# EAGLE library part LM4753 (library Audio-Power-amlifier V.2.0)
The LM4753 is a stereo audio amplifier capable of delivering 10W/channel at 10% distortion into a 8W load. The power amp has an internally set gain of 30 dB. A 0V–5V DC controlled volume block provides 80 dB of attenuation from input to line-out. Line outputs are available after the volume control for signal routing.
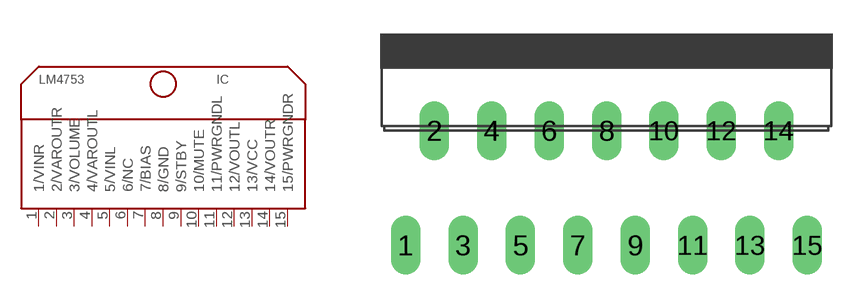
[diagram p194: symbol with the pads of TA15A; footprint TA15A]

Designator prefix IC

## LM4753  [TA15A]
1  1/VINR  in
2  2/VAROUTR  out
3  3/VOLUME  in
4  4/VAROUTL  out
5  5/VINL  in
6  6/NC  nc
7  7/BIAS
8  8/GND  pwr
9  9/STBY  in
10  10/MUTE  in
11  11/PWRGNDL  pwr
12  12/VOUTL  out
13  13/VCC  pwr
14  14/VOUTR  out
15  15/PWRGNDR  pwr

## Footprint TA15A (pad centres in mm)
TA15A www.national.com
drill 0.8 long: 1 -8.89,-5.08; 2 -7.62,0; 3 -6.35,-5.08; 4 -5.08,0; 5 -3.81,-5.08; 6 -2.54,0; 7 -1.27,-5.08; 8 0,0; 9 1.27,-5.08; 10 2.54,0; 11 3.81,-5.08; 12 5.08,0; 13 6.35,-5.08; 14 7.62,0; 15 8.89,-5.08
